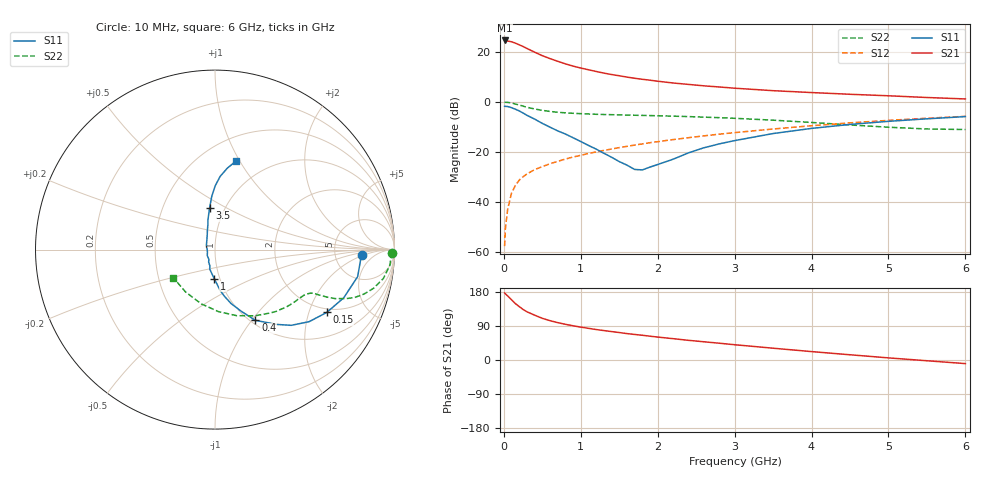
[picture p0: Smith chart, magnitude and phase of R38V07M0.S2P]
! SIEMENS Small Signal Semiconductors
! BFR181
! Si NPN RF Bipolar Junction Transistor in SOT23
! VCE = 8 V  IC = 7 mA
! Common Emitter S-Parameters:  May  1996
# GHz  S  MA  R  50
!  f  S11  S21  S12  S22
! GHz  MAG  ANG  MAG  ANG  MAG  ANG  MAG  ANG
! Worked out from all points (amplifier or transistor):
!   36 points, 10 MHz to 6 GHz, reference 50 ohm
!   highest |S21| = 24.6 dB at 10 MHz (marker M1)
!   |S21| within 3 dB of that: start of sweep to 287.8 MHz
!   unconditionally stable (mu >= 1): 1.041 GHz to 2.98 GHz
!   at 250 MHz: K = 0.49, MSG = 26.1 dB, |S12| = -30.0 dB
!   at 1.4 GHz: K = 1.04, MAG = 13.6 dB, |S12| = -18.9 dB
!   at 6 GHz: K = 0.86, MSG = 3.5 dB, |S12| = -5.8 dB
!   S11 on the Smith chart (normalised r, x): 10 MHz: 9.58, -1.81; 150 MHz: 1.85, -2.65; 400 MHz: 1.05, -1.04; 1 GHz: 0.94, -0.31; 3.5 GHz: 0.85, +0.41; 6 GHz: 0.73, +0.97
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0.01  0.8169 -2.2  16.96 176.9  0.0013 91.5  0.9878 -1.0
0.02  0.8129 -4.2  16.86 174.7  0.0029 87.6  0.9825 -2.1
0.05  0.8091 -10.7  16.55 169.0  0.0072 86.1  0.9782 -5.1
0.1  0.766 -20.5  15.95 159.0  0.015 80.0  0.952 -9.7
0.15  0.7147 -29.3  14.97 148.8  0.0214 74.2  0.9081 -13.8
0.2  0.6607 -37.4  13.88 141.0  0.0272 72.1  0.8665 -16.6
0.25  0.5989 -44.8  12.84 133.4  0.0318 69.1  0.8231 -18.9
0.3  0.5393 -50.6  11.75 127.3  0.0362 68.9  0.7824 -20.4
0.4  0.4536 -60.3  9.894 118.3  0.0442 66.7  0.7225 -22.2
0.5  0.3718 -67.1  8.411 110.0  0.0508 66.6  0.6773 -23.0
0.6  0.3126 -73.5  7.356 103.8  0.0579 66.0  0.6444 -23.4
0.7  0.2632 -78.8  6.496 98.6  0.0647 66.5  0.6209 -23.7
0.8  0.2281 -83.0  5.775 94.2  0.0718 66.5  0.604 -23.8
1  0.1615 -91.6  4.761 86.8  0.0854 66.7  0.582 -24.7
1.1  0.1347 -97.5  4.397 83.6  0.0929 66.8  0.5735 -25.4
1.6  0.0544 -142.6  3.139 69.7  0.1291 66.1  0.5458 -29.4
1.8  0.0436 178.5  2.836 65.3  0.1446 65.3  0.537 -31.5
2.2  0.0714 129.2  2.391 56.3  0.1764 63.3  0.5189 -36.4
3.5  0.2329 97.5  1.678 31.1  0.2872 53.5  0.4312 -58.8
4.5  0.3545 89.9  1.421 13.8  0.3809 43.2  0.346 -86.8
5.5  0.459 81.4  1.225 -2.0  0.4716 31.0  0.2874 -124.8
6  0.5083 76.5  1.146 -9.5  0.5142 24.2  0.2803 -146.3
